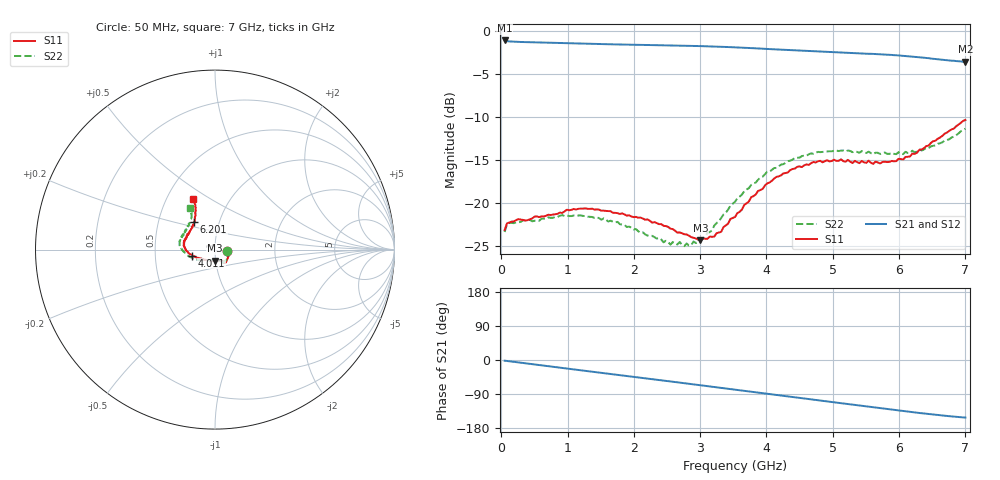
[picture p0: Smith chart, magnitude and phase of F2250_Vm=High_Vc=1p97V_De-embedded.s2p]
! Integrated Device Technology
! Corporate Headquarters
! 6024 Silver Creek Valley Road
! San Jose, CA 95138  USA
! Phone:  1-408-284-8200
! Toll Free:  1-800-223-1366
! Webpage:  http://www.idt.com/
! Timing and RF Division
! 515 Groton Road, Suite 102
! Westford, MA 01886-6024
! Device:  F2250
! Description: Voltage Variable RF Attenuator
! Frequency:  50.0 -  6000.00 MHz
! Package:  3x3 mm Thin QFN Plastic Package: 16 pin
! Ports:  2 RF, 3 DC
!  Pin  1  = GND
!  Pin  2  = NC
!  Pin  3  = RF1  = Port 1
!  Pin  4  = NC
!  Pin  5  = GND
!  Pin  6  = GND
!  Pin  7  = GND
!  Pin  8  = GND
!  Pin  9  = NC
!  Pin 10  = RF2  = Port 2
!  Pin 11  = NC
!  Pin 12  = GND
!  Pin 13  = GND
!  Pin 14  = VCNTRL
!  Pin 15  = VDD
!  Pin 16  = VMODE
! Vcntrl:  1.970 Volts
! Vmode:  +3.300 Volts
! Vdd:  +3.30  Volts
! Current:  1.321 mA
! Data:  The device was measured on a the F2250 evaluation board which has
!  individual transmission lines to the RF pins.  Data was collected
!  using a calibrated network analyzer.  The evaluation board was
!  de-embedded using a TRL calibration technique.
!  The reference plane is the edge of the package pin.
! Misc:  SN 10
!  Action Tracker AT0258
! Date Measured:  2014-11-26
! Date:  2015-10-15  MJV
! Note:
!  Integrated Device Technology supplies this data as a sample of measured
!  data at the package pin for this product.  Your particular data for this
!  product may vary.
!  Data was taken at 25 degrees C.
!  Integrated Device Technology reserves the right to change this data at anytime.
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# GHz S dB R 50
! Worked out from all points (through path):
!   201 points, 50 MHz to 7 GHz, reference 50 ohm
!   highest |S21| = -1.06 dB at 50 MHz (marker M1); lowest = -3.5 dB at 7 GHz (marker M2)
!   group delay of S21, straight-line fit = 61.1 ps
!   lowest |S11| = -24.3 dB at 3.004 GHz (marker M3), VSWR 1.13, Z = 49.6 - j6.07 ohm
!   |S11| at or under -10 dB: start of sweep to end of sweep
!   |S22| runs from -25.0 to -11.3 dB; largest |S21 - S12| = 0.0019
!   S11 on the Smith chart (normalised r, x): 50 MHz: 1.15, -0.02; 4.011 GHz: 0.77, -0.05; 6.201 GHz: 0.76, +0.24; 7 GHz: 0.68, +0.42
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0.05  -23.12 -8.1  -1.06 -1.8  -1.06 -1.8  -23.33 -8.9
0.08475  -22.35 -7.5  -1.14 -2.5  -1.14 -2.5  -22.47 -8.0
0.1195  -22.23 -8.1  -1.17 -3.3  -1.17 -3.3  -22.30 -7.7
0.6755  -21.45 -31.7  -1.32 -15.7  -1.32 -15.7  -21.80 -33.6
1.2315  -20.63 -50.2  -1.44 -27.9  -1.43 -27.9  -21.47 -56.7
1.75275  -21.14 -57.1  -1.53 -39.1  -1.53 -39.1  -22.16 -65.1
2.37825  -22.42 -58.3  -1.62 -52.7  -1.62 -52.7  -24.04 -70.2
2.552  -22.96 -62.3  -1.64 -56.6  -1.64 -56.6  -24.80 -76.7
2.691  -23.39 -68.5  -1.66 -59.7  -1.66 -59.7  -24.50 -83.4
2.7605  -23.60 -70.3  -1.67 -61.2  -1.68 -61.2  -24.99 -87.5
3.00375  -24.30 -90.2  -1.72 -66.7  -1.72 -66.7  -24.09 -108.0
3.21225  -23.87 -111.1  -1.77 -71.4  -1.77 -71.4  -22.60 -125.7
3.525  -21.60 -139.7  -1.86 -78.5  -1.86 -78.5  -19.82 -144.6
3.76825  -19.30 -155.2  -1.95 -84.0  -1.95 -84.0  -17.87 -156.2
4.0115  -17.68 -165.3  -2.05 -89.4  -2.05 -89.4  -16.33 -166.1
4.4285  -15.97 -177.9  -2.21 -98.6  -2.22 -98.6  -14.72 -179.0
4.7065  -15.20 174.6  -2.31 -104.8  -2.31 -104.8  -14.24 174.9
5.054  -15.06 166.3  -2.44 -112.4  -2.44 -112.5  -13.85 167.6
5.85325  -15.18 139.7  -2.74 -129.9  -2.74 -130.0  -14.26 148.4
6.20075  -14.22 127.3  -2.94 -137.6  -2.95 -137.7  -13.88 139.2
6.54825  -12.72 118.6  -3.21 -144.6  -3.22 -144.8  -13.28 127.7
7  -10.31 113.1  -3.54 -152.0  -3.55 -152.1  -11.33 121.3
